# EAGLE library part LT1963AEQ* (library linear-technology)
LT1963 1.5A, Low Noise, Fast Transient Response LDO Regulator Source: http://www.linear.com
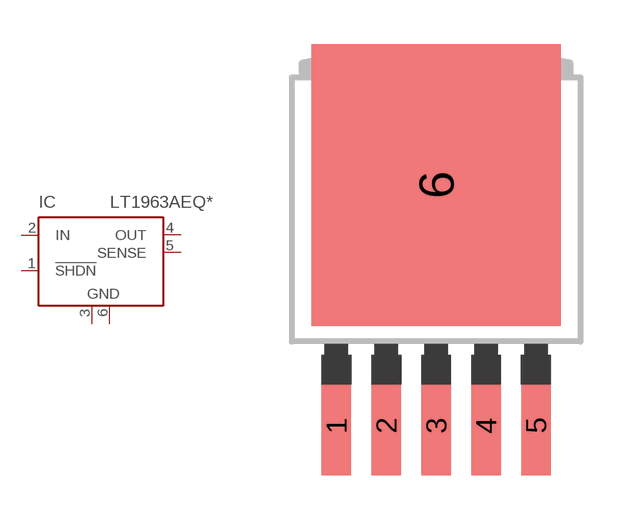
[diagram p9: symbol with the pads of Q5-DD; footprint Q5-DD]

Designator prefix IC

## LT1963AEQ (MPN: LT1963AEQ; OC_FARNELL: 1273625; OC_NEWARK: 57M7427), LT1963AEQ-1.5 (MPN: LT1963AEQ-1.5; OC_FARNELL: unknown; OC_NEWARK: 57M7428), LT1963AEQ-1.8 (MPN: LT1963AEQ-1.8; OC_FARNELL: 1663522; OC_NEWARK: 57M7432), LT1963AEQ-2.5 (MPN: LT1963AEQ-2.5; OC_FARNELL: 1500530; OC_NEWARK: 53K8985), LT1963AEQ-3.3 (MPN: LT1963AEQ-3.3; OC_FARNELL: 1273626; OC_NEWARK: 57M7439)  [Q5-DD]
1  !SHDN  in
2  IN  in
3  GND  pwr
4  OUT  pas
5  SENSE  in
6  GND  pwr

## Footprint Q5-DD (pad centres in mm)
Q5-DD
smd 1 x 3.4: 1 -3.4,-7.875; 2 -1.7,-7.875; 3 0,-7.875; 4 1.7,-7.875; 5 3.4,-7.875
smd 8.5 x 9.6: 6 0,0.325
